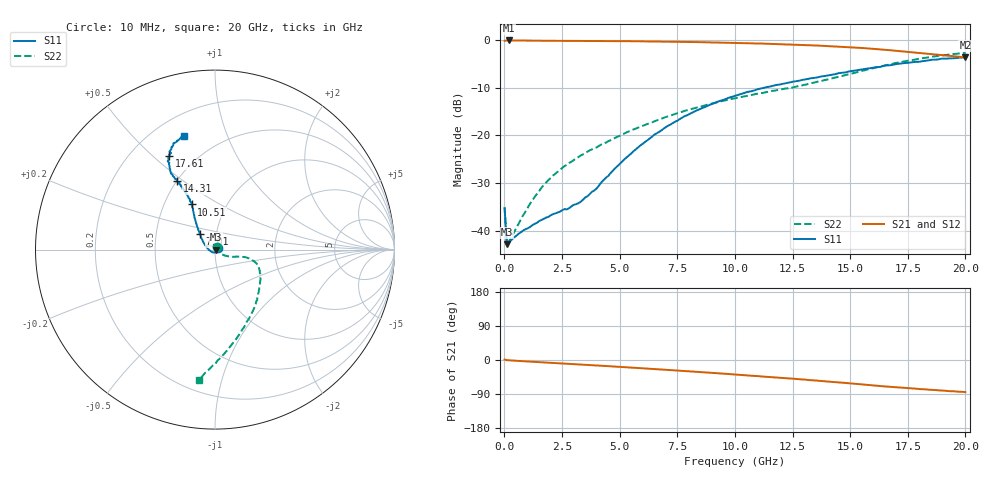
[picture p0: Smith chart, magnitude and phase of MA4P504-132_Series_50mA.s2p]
! AWR Design Environment (9226) Thu Aug 19 02:45:16 2021
! Document = '50mA'
! nPorts: 2, nXvals: 201
# GHz S DB R 50
!Freq DBS11 AngS11 DBS21 AngS21 DBS12 AngS12 DBS22 AngS22
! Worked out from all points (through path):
!   201 points, 10 MHz to 20 GHz, reference 50 ohm
!   highest |S21| = -0.11 dB at 210 MHz (marker M1); lowest = -3.7 dB at 20 GHz (marker M2)
!   group delay of S21, straight-line fit = 12 ps
!   lowest |S11| = -42.9 dB at 110 MHz (marker M3), VSWR 1.01, Z = 50.7 + j0.027 ohm
!   |S11| at or under -10 dB: start of sweep to 11.3 GHz
!   |S22| runs from -43.3 to -2.7 dB; largest |S21 - S12| = 0.031
!   S11 on the Smith chart (normalised r, x): 10 MHz: 1.03, +0.01; 7.01 GHz: 0.83, +0.15; 10.51 GHz: 0.69, +0.38; 14.31 GHz: 0.50, +0.47; 17.61 GHz: 0.36, +0.57; 20 GHz: 0.32, +0.71
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0.01  -35.39 24.6  -0.19 1.2  -0.13 0.3  -35.07 49.4
0.11  -42.89 2.1  -0.12 -0.4  -0.10 -0.5  -43.28 0.2
0.21  -42.39 -0.3  -0.11 -0.9  -0.11 -0.9  -42.12 0.4
1.11  -39.26 -34.3  -0.15 -4.3  -0.14 -4.2  -34.39 -23.4
1.61  -37.78 -55.3  -0.17 -6.1  -0.16 -5.9  -31.01 -28.8
2.61  -35.51 -101.6  -0.20 -9.6  -0.19 -9.2  -26.46 -33.4
2.71  -35.55 -106.0  -0.20 -9.9  -0.19 -9.6  -26.21 -32.7
3.41  -33.52 -140.8  -0.22 -12.4  -0.21 -12.0  -24.00 -31.1
4.01  -31.14 -166.6  -0.23 -14.5  -0.22 -14.1  -22.55 -28.4
5.21  -25.03 158.8  -0.26 -18.9  -0.25 -18.3  -19.63 -22.6
6.71  -19.31 137.0  -0.32 -24.7  -0.32 -23.9  -16.74 -15.8
7.01  -18.28 134.3  -0.34 -25.8  -0.34 -25.1  -16.18 -15.2
8.31  -14.87 125.6  -0.45 -31.1  -0.45 -30.1  -14.24 -14.5
10.01  -11.75 118.2  -0.62 -38.3  -0.62 -36.9  -12.26 -18.4
10.51  -10.97 117.3  -0.69 -40.4  -0.67 -38.9  -11.77 -21.1
12.01  -9.29 116.8  -0.91 -47.1  -0.84 -45.4  -10.37 -33.2
13.41  -7.99 118.2  -1.14 -53.6  -1.06 -52.1  -8.97 -48.1
14.31  -7.22 119.2  -1.36 -58.1  -1.24 -56.6  -7.94 -58.1
16.71  -5.33 118.2  -2.15 -70.6  -2.04 -69.2  -5.14 -81.8
17.61  -4.74 116.0  -2.54 -74.8  -2.45 -73.9  -4.27 -87.9
19.01  -3.93 111.3  -3.16 -80.6  -3.18 -80.4  -3.25 -94.5
20  -3.65 105.2  -3.67 -84.8  -3.77 -84.2  -2.71 -96.8
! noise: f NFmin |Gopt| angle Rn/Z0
0.01  0  1  0  2e-20
2.21  0  1  0  2e-20
4.41  0  1  0  2e-20
6.61  0  1  0  2e-20
8.81  0  1  0  2e-20
11.11  0  1  0  2e-20
13.31  0  1  0  2e-20
15.51  0  1  0  2e-20
17.71  0  1  0  2e-20
20  0  1  0  2e-20
